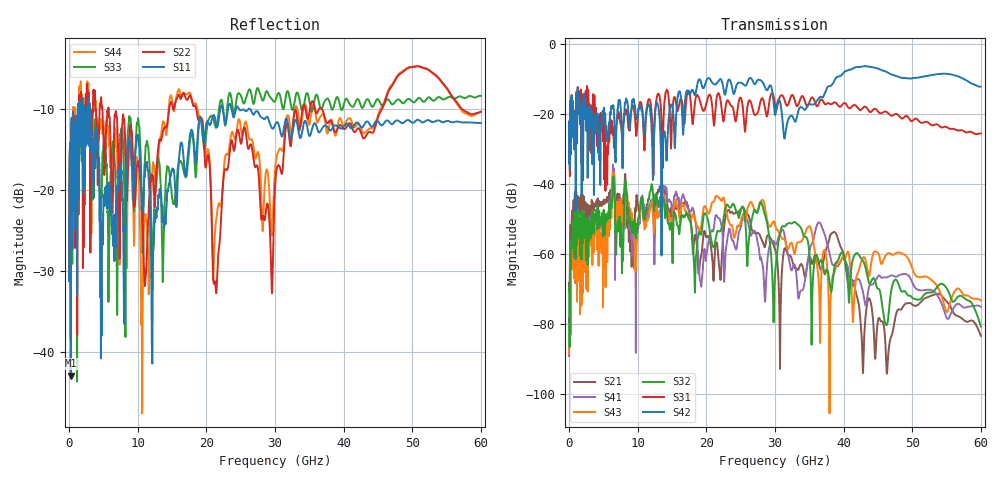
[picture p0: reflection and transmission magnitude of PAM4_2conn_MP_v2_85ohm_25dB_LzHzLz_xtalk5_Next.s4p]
! Info: Touchstone file created by Circ.  Input file=FAB50GbE_2conn_Midplane_Examax_Topo2_v2_85ohm_25dB_LzHzLz.circ
# Hz S RI R 50
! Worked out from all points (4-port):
!   6000 points, 10 MHz to 60 GHz, reference 50 ohm
!   strongest paths, dB at 10 MHz, 15.01 GHz, 30.01 GHz, 45.01 GHz, 60 GHz:
!     S42: -34.0, -17.4, -20.2, -7.0, -12.1
!     S31: -34.0, -20.9, -17.2, -19.2, -25.5
!     S32: -70.0, -55.5, -65.9, -69.8, -80.6
!     S43: -88.4, -51.8, -51.4, -59.6, -73.2
!     S41: -89.1, -47.6, -57.0, -66.3, -75.0
!     S21: -69.7, -51.3, -58.6, -78.9, -83.3
!   lowest |S11| = -42.9 dB at 260 MHz (marker M1), VSWR 1.01, Z = 50.1 + j0.712 ohm
!   |S11| at or under -10 dB: 3.064 GHz to 22.01 GHz (18.94 GHz wide, 151 % of centre); 24.8 GHz to 26.07 GHz (1.275 GHz wide, 5.01 % of centre); 26.43 GHz to end of sweep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
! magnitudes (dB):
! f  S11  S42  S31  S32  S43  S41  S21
! 10 MHz  -31.2  -34.0  -34.0  -70.0  -88.4  -89.1  -69.7
! 260 MHz  -42.9  -23.2  -22.2  -60.5  -69.3  -62.8  -54.0
! 6.35 GHz  -23.8  -17.9  -25.9  -41.5  -38.2  -36.4  -39.8
! 10.64 GHz  -22.5  -18.9  -18.3  -43.9  -44.7  -43.3  -44.8
! 19.22 GHz  -11.3  -10.8  -17.2  -54.3  -52.8  -68.9  -60.5
! 21.29 GHz  -11.1  -11.5  -19.7  -56.3  -43.9  -49.4  -58.0
! 60 GHz  -11.7  -12.1  -25.5  -80.6  -73.2  -75.0  -83.3
